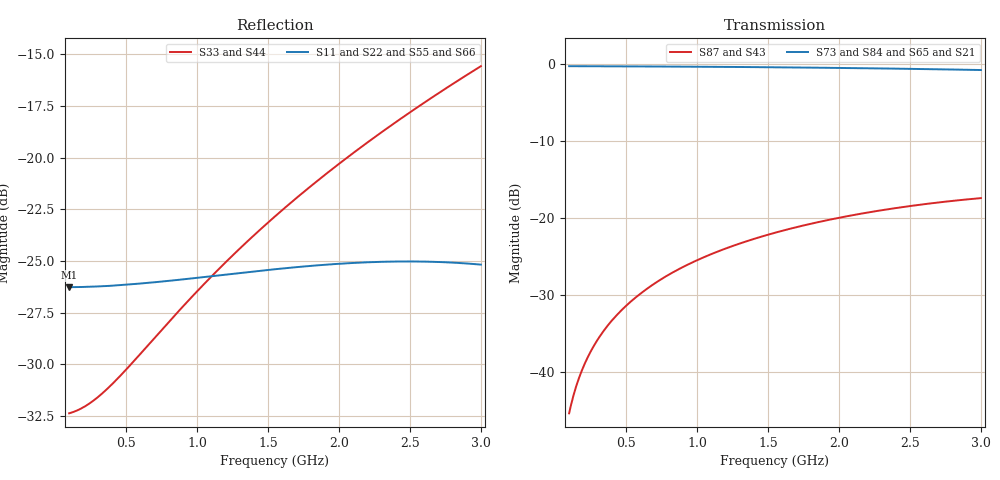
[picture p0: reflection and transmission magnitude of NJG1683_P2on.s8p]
! Created Wed May 22 11:48:50 2013
# hz S ma R 50
! 8 Port Network Data from SP2.SP block
! freq  magS11  angS11  magS12  angS12  magS13  angS13  magS14  angS14
!  magS15  angS15  magS16  angS16  magS17  angS17  magS18  angS18
!  magS21  angS21  magS22  angS22  magS23  angS23  magS24  angS24
!  magS25  angS25  magS26  angS26  magS27  angS27  magS28  angS28
!  magS31  angS31  magS32  angS32  magS33  angS33  magS34  angS34
!  magS35  angS35  magS36  angS36  magS37  angS37  magS38  angS38
!  magS41  angS41  magS42  angS42  magS43  angS43  magS44  angS44
!  magS45  angS45  magS46  angS46  magS47  angS47  magS48  angS48
!  magS51  angS51  magS52  angS52  magS53  angS53  magS54  angS54
!  magS55  angS55  magS56  angS56  magS57  angS57  magS58  angS58
!  magS61  angS61  magS62  angS62  magS63  angS63  magS64  angS64
!  magS65  angS65  magS66  angS66  magS67  angS67  magS68  angS68
!  magS71  angS71  magS72  angS72  magS73  angS73  magS74  angS74
!  magS75  angS75  magS76  angS76  magS77  angS77  magS78  angS78
!  magS81  angS81  magS82  angS82  magS83  angS83  magS84  angS84
!  magS85  angS85  magS86  angS86  magS87  angS87  magS88  angS88
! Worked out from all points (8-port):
!   291 points, 100 MHz to 3 GHz, reference 50 ohm
!   strongest paths, dB at 100 MHz, 820 MHz, 1.55 GHz, 2.28 GHz, 3 GHz:
!     S73: -0.3, -0.3, -0.4, -0.5, -0.8
!     S84: -0.3, -0.3, -0.4, -0.6, -0.8
!     S65: -0.5, -0.5, -0.5, -0.6, -0.6
!     S21: -0.5, -0.5, -0.5, -0.6, -0.6
!     S87: -45.4, -27.2, -21.9, -19.0, -17.4
!     S43: -45.4, -27.2, -22.0, -19.2, -17.6
!   lowest |S11| = -26.3 dB at 100 MHz (marker M1), VSWR 1.10, Z = 55.1 + j0.127 ohm
!   |S11| at or under -10 dB: start of sweep to end of sweep
